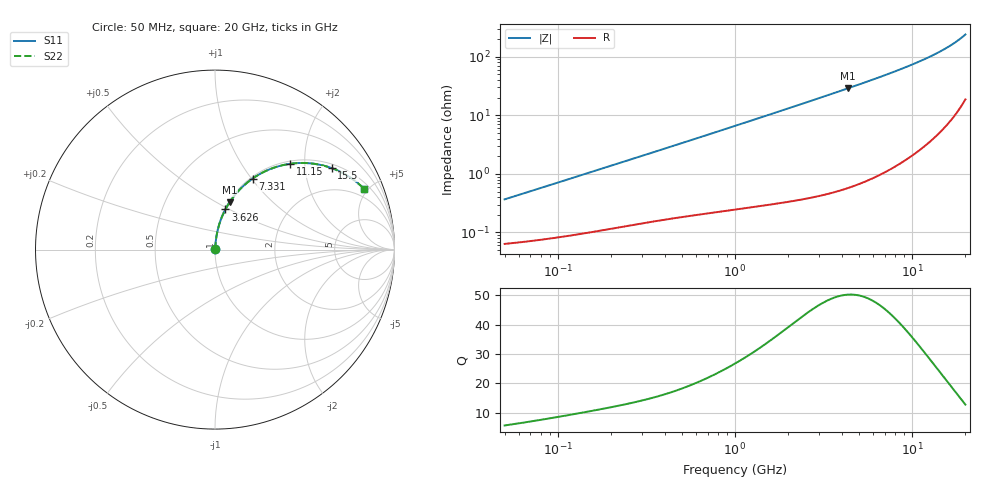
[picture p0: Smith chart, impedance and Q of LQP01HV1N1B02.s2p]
!Murata Part Number: LQP01HV1N1B02
!These Parameters are Measured in Series Mode Connection
!  o--[Z]--o
!Port1  Port2
!  o-------o
!Freq. Start=50[MHz] Stop=20[GHz], 401[Steps]
# Hz S RI R 50
!Freq.(Hz) S11(Real) S11(Imag) S21(Real) S21(Imag) S12(Real) S12(Imag) S22(Real) S22(Imag)
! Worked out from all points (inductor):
!   401 points, 50 MHz to 20 GHz, reference 50 ohm
!   read as one part in series: L = 1.14 nH near 51.52 MHz
!   highest Q = 50.3 at 4.34 GHz (marker M1), where L = 1.06 nH
!   S11 on the Smith chart (normalised r, x): 50 MHz: 1.00, +0.01; 3.626 GHz: 1.01, +0.48; 7.331 GHz: 1.02, +1.01; 11.15 GHz: 1.05, +1.68; 15.5 GHz: 1.13, +2.77; 20 GHz: 1.37, +4.76
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5e7  0.000651 0.00361  0.9993 -0.00361  0.9993 -0.00361  0.000651 0.00361
5.152053e7  0.000657 0.00372  0.9993 -0.00372  0.9993 -0.00372  0.000657 0.00372
1.364002e8  0.00104 0.0095  0.999 -0.0095  0.999 -0.0095  0.00104 0.0095
3.721004e8  0.00222 0.025  0.9978 -0.025  0.9978 -0.025  0.00222 0.025
6.380365e8  0.00381 0.0421  0.9962 -0.0421  0.9962 -0.0421  0.00381 0.0421
1e9  0.00673 0.0652  0.9933 -0.0652  0.9933 -0.0652  0.00673 0.0652
1.714689e9  0.0154 0.1102  0.9846 -0.1102  0.9846 -0.1102  0.0154 0.1102
2.728004e9  0.0346 0.172  0.9654 -0.172  0.9654 -0.172  0.0346 0.172
3.626126e9  0.0581 0.224  0.9419 -0.224  0.9419 -0.224  0.0581 0.224
4.34015e9  0.0809 0.263  0.9191 -0.263  0.9191 -0.263  0.0809 0.263
5.769027e9  0.1364 0.3331  0.8636 -0.3331  0.8636 -0.3331  0.1364 0.3331
7.331367e9  0.2094 0.3958  0.7906 -0.3958  0.7906 -0.3958  0.2094 0.3958
7.442007e9  0.2149 0.3996  0.7851 -0.3996  0.7851 -0.3996  0.2149 0.3996
9.178299e9  0.307 0.4484  0.693 -0.4484  0.693 -0.4484  0.307 0.4484
1.115139e10  0.4177 0.4779  0.5823 -0.4779  0.5823 -0.4779  0.4177 0.4779
1.220001e10  0.4768 0.4827  0.5232 -0.4827  0.5232 -0.4827  0.4768 0.4827
1.334722e10  0.5399 0.4798  0.4601 -0.4798  0.4601 -0.4798  0.5399 0.4798
1.438523e10  0.5949 0.4704  0.4051 -0.4704  0.4051 -0.4704  0.5949 0.4704
1.550395e10  0.651 0.4538  0.349 -0.4538  0.349 -0.4538  0.651 0.4538
1.747767e10  0.74 0.4106  0.26 -0.4106  0.26 -0.4106  0.74 0.4106
1.940974e10  0.8131 0.3552  0.1869 -0.3552  0.1869 -0.3552  0.8131 0.3552
2e10  0.8325 0.3364  0.1675 -0.3364  0.1675 -0.3364  0.8325 0.3364
